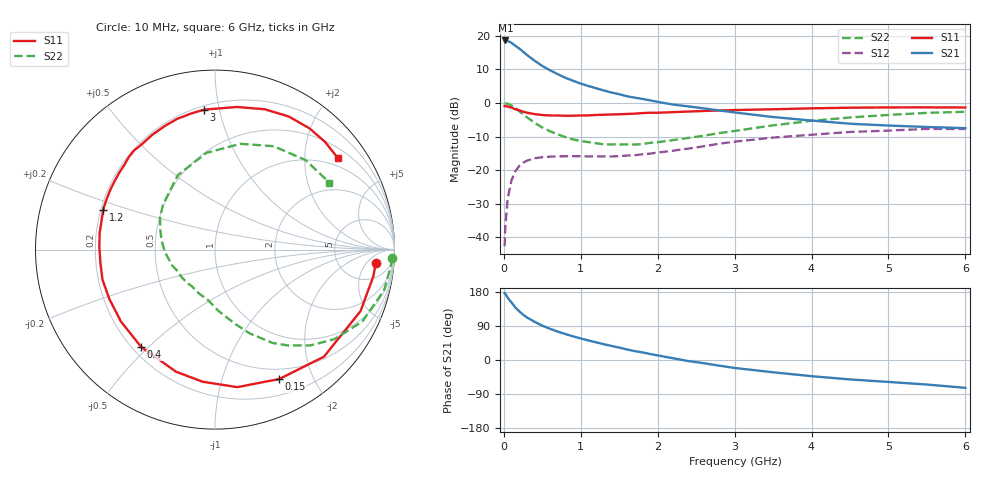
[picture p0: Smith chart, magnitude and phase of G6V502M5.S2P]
! SIEMENS Small Signal Semiconductors
! BFG193
! Si NPN RF Bipolar Junction Transistor in SOT223
! VCE = 0.5 V  IC = 2.5 mA
! Common Emitter S-Parameters:  August  1996
# GHz  S  MA  R  50
!  f  S11  S21  S12  S22
! GHz  MAG  ANG  MAG  ANG  MAG  ANG  MAG  ANG
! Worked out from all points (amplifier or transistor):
!   36 points, 10 MHz to 6 GHz, reference 50 ohm
!   highest |S21| = 18.6 dB at 20 MHz (marker M1)
!   |S21| within 3 dB of that: start of sweep to 232.1 MHz
!   unconditionally stable (mu >= 1): 1.245 GHz to end of sweep
!   at 250 MHz: K = 0.23, MSG = 16.5 dB, |S12| = -17.8 dB
!   at 1.4 GHz: K = 1.10, MAG = 7.6 dB, |S12| = -15.9 dB
!   at 6 GHz: K = 1.03, MAG = -0.9 dB, |S12| = -7.8 dB
!   S11 on the Smith chart (normalised r, x): 10 MHz: 12, -9; 150 MHz: 0.38, -1.55; 400 MHz: 0.23, -0.48; 1.2 GHz: 0.21, +0.17; 3 GHz: 0.22, +0.90; 6 GHz: 0.75, +2.82
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0.01  0.8982 -4.7  8.464 176.8  0.0074 89.8  0.989 -2.8
0.02  0.8951 -9.5  8.478 174.7  0.0149 86.9  0.9837 -5.5
0.05  0.8804 -22.9  8.301 164.3  0.0378 76.2  0.9688 -13.6
0.1  0.851 -44.5  7.82 151.8  0.0709 65.8  0.9137 -26.0
0.15  0.805 -63.6  7.063 138.5  0.0964 54.8  0.8313 -36.9
0.2  0.7763 -80.8  6.438 128.8  0.1152 47.4  0.7544 -45.0
0.25  0.7393 -95.4  5.771 119.6  0.1288 40.5  0.6725 -52.6
0.3  0.7142 -107.7  5.17 112.3  0.1382 35.6  0.6115 -58.3
0.4  0.6809 -127.1  4.241 100.7  0.15 27.6  0.5055 -67.5
0.5  0.6597 -142.6  3.539 90.6  0.1556 21.8  0.4301 -74.7
0.6  0.6498 -154.9  3.056 82.4  0.1587 18.4  0.3787 -80.8
0.7  0.6489 -165.0  2.675 75.0  0.1601 15.5  0.3411 -86.9
0.9  0.6445 178.8  2.133 62.4  0.1613 12.0  0.2861 -97.3
1.1  0.6517 166.3  1.78 51.6  0.1601 10.4  0.2608 -109.6
1.2  0.6617 160.3  1.65 46.6  0.1597 10.2  0.2516 -115.5
1.6  0.6845 141.0  1.256 27.8  0.1648 11.3  0.2415 -140.6
2.2  0.7284 118.8  0.944 4.6  0.1945 12.5  0.2795 -177.1
3  0.7822 94.4  0.721 -21.0  0.2652 5.1  0.3822 139.4
3.5  0.8038 81.3  0.616 -32.4  0.3048 -5.7  0.4637 116.5
4.5  0.8479 61.0  0.49 -51.3  0.3695 -24.9  0.6062 76.5
5.5  0.8578 44.4  0.438 -64.8  0.4101 -48.3  0.71 44.6
6  0.8537 36.9  0.421 -73.4  0.4095 -61.4  0.7379 30.4
